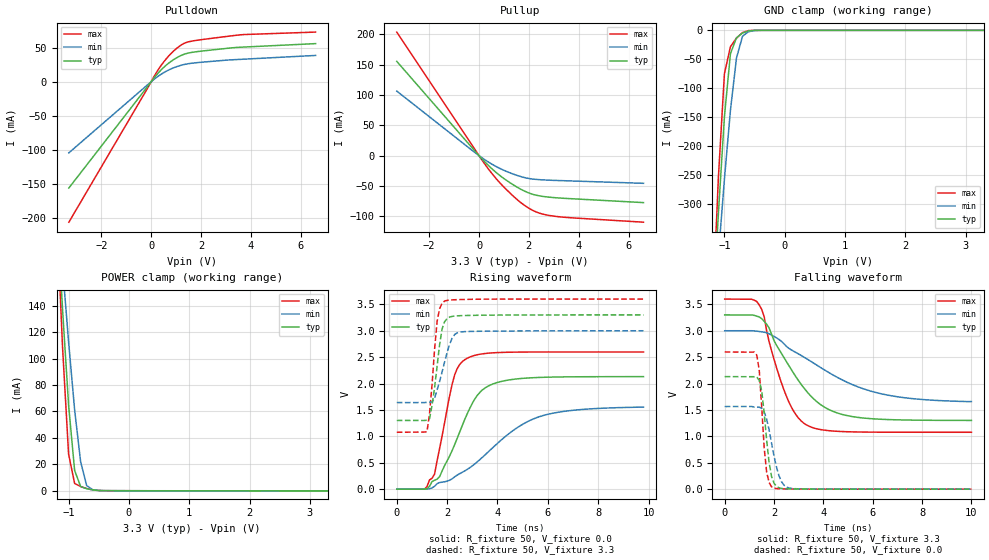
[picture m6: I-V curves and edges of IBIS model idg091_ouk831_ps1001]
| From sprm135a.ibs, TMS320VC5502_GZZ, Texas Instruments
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[Model]   idg091_ouk831_ps1001
Model_type   I/O
Vinh = 2.00
Vinl = 0.80
Enable   Active-Low
Polarity   Non-Inverting
| signals   A, GZ, Y
Vmeas = 1.5
|   typ   min   max
C_comp   1.997p   1.996p   1.999p
|   typ   min   max
[Temperature Range]   25   -40   125
|   typ   min   max
[Voltage Range]   3.30V   3.00V   3.60V
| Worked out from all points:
|   slope of the pulldown table from 0 to 0.495 V, typ, clamps not added: 24 ohm
|   slope of the pullup table from 0 to 0.495 V, typ, clamps not added: 23.8 ohm
|   GND clamp passes 1 mA (typ) near -0.60 V on its own axis
|   POWER clamp passes 1 mA (typ) near -0.64 V on its own axis
|   rising waveform, R_fixture 50, V_fixture 0.0: 20-80 % time 1.22ns typ, 2.49ns min, 657ps max; typ from 0 V to 2.13 V
|   falling waveform, R_fixture 50, V_fixture 3.3: 20-80 % time 1.7ns typ, 3.02ns min, 1.01ns max; typ from 3.3 V to 1.3 V
|   rising waveform, R_fixture 50, V_fixture 3.3: 20-80 % time 320ps typ, 466ps min, 257ps max; typ from 1.3 V to 3.3 V
|   falling waveform, R_fixture 50, V_fixture 0.0: 20-80 % time 292ps typ, 428ps min, 232ps max; typ from 2.13 V to 0 V
[Pulldown]
|   Voltage   I(typ)   I(min)   I(max)
-3.3V     -155.6mA   -104.1mA   -205.6mA
200mV     9.243mA    5.866mA    12.7mA
600mV     24.13mA    15.28mA    33.3mA
800mV     29.87mA    18.87mA    41.37mA
1.1V      36.63mA    23.02mA    51.08mA
1.3V      39.97mA    25.04mA    55.82mA
1.6V      42.83mA    27mA       59.29mA
3.5V      50.44mA    32.65mA    68.4mA
6.6V      55.87mA    38.54mA    72.75mA
[GND_clamp]
|   Voltage   I(typ)   I(min)   I(max)
-3.3V     -4.925A    -3.709A    -6.397A
-1.2V     -505.2mA   -529.5mA   -496.9mA
-1.1V     -317.2mA   -390.3mA   -254.5mA
-1V       -149.6mA   -257.7mA   -75.06mA
-900mV    -40.21mA   -138.1mA   -28.26mA
-800mV    -12.98mA   -47.92mA   -13.48mA
-700mV    -4.668mA   -10.2mA    -3.929mA
-600mV    -901.5uA   -2.361mA   -447.5uA
-400mV    -4.618uA   -50.5uA    -472.2nA
3.3V      444.1pA    1.932uA    266.4pA
[Pullup]
|   Voltage   I(typ)   I(min)   I(max)
-3.3V     155.5mA    106.5mA    203.9mA
-200mV    9.306mA    6.233mA    12.42mA
300mV     -13.07mA   -8.546mA   -17.75mA
600mV     -24.68mA   -16mA      -33.65mA
900mV     -34.78mA   -22.33mA   -47.64mA
1.4V      -48.81mA   -30.78mA   -67.77mA
1.7V      -55.9mA    -34.78mA   -78.19mA
2V        -61.53mA   -37.68mA   -86.71mA
2.3V      -65.31mA   -39.22mA   -93.01mA
2.9V      -68.83mA   -40.61mA   -99.22mA
3.7V      -71.03mA   -41.73mA   -102.5mA
6.6V      -77.46mA   -45.65mA   -109.8mA
[POWER_clamp]
|   Voltage   I(typ)   I(min)   I(max)
-3.3V     2.112A     1.593A     2.741A
-1.2V     218.1mA    229.3mA    213.2mA
-1.1V     137.3mA    169.6mA    108.5mA
-1V       64.88mA    112.7mA    27.71mA
-900mV    15.37mA    61.29mA    5.523mA
-800mV    3.157mA    21.76mA    3.151mA
-700mV    1.498mA    3.887mA    1.661mA
-600mV    649.7uA    748uA      624uA
-500mV    185.1uA    179.4uA    140.5uA
3.3V      -108.3uA   -68.12uA   -162.1uA
[Ramp]
|   I(typ)   I(min)   I(max)
dV/dt_r   1.278/1.218n   0.933/2.489n   1.559/0.652n
dV/dt_f   1.199/1.700n   0.806/3.024n   1.513/1.007n
[Rising Waveform]
R_fixture = 50
V_fixture = 0.0
|  pu_on
|  TIME   V(typ)   V(min)   V(max)
0s        5nV        18nV       4nV
1.1ns     50.37uV    -132uV     2.228mV
1.5ns     168.6mV    53.81mV    283.9mV
1.7ns     236mV      125mV      767.4mV
2.3ns     844.2mV    233.6mV    2.165V
2.8ns     1.429V     374.8mV    2.48V
3.2ns     1.777V     518.3mV    2.546V
3.7ns     1.968V     735.7mV    2.578V
5.6ns     2.115V     1.362V     2.597V
9.8ns     2.131V     1.554V     2.598V
[Falling Waveform]
R_fixture = 50
V_fixture = 3.3
V_fixture_min = 3.0
V_fixture_max = 3.6
|  pd_on
|  TIME   V(typ)   V(min)   V(max)
0s        3.3V       3V         3.6V
1.4ns     3.262V     2.986V     3.489V
1.6ns     3.179V     2.973V     3.268V
1.8ns     3.053V     2.942V     2.794V
2.5ns     2.417V     2.706V     1.761V
3.3ns     1.865V     2.476V     1.22V
4.1ns     1.538V     2.242V     1.114V
5.1ns     1.381V     1.995V     1.086V
7ns       1.313V     1.75V      1.078V
10ns      1.302V     1.659V     1.078V
[Rising Waveform]
R_fixture = 50
V_fixture = 3.3
V_fixture_min = 3.0
V_fixture_max = 3.6
|  pd_off
|  TIME   V(typ)   V(min)   V(max)
0s        1.301V     1.64V      1.078V
1.2ns     1.306V     1.644V     1.087V
1.3ns     1.333V     1.649V     1.429V
1.4ns     1.585V     1.648V     1.973V
1.6ns     2.321V     1.877V     3.172V
1.8ns     3.033V     2.218V     3.524V
1.9ns     3.172V     2.408V     3.562V
2.2ns     3.272V     2.86V      3.584V
2.5ns     3.285V     2.973V     3.591V
9.8ns     3.3V       3V         3.6V
[Falling Waveform]
R_fixture = 50
V_fixture = 0.0
|  pu_off
|  TIME   V(typ)   V(min)   V(max)
0s        2.131V     1.565V     2.598V
1.3ns     2.126V     1.554V     2.539V
1.4ns     2.059V     1.552V     2.255V
1.5ns     1.86V      1.531V     1.558V
1.6ns     1.446V     1.464V     786.2mV
1.7ns     930.2mV    1.329V     323.7mV
1.9ns     239.4mV    870.1mV    44.48mV
2.2ns     26.16mV    256.8mV    7.89mV
2.6ns     6.345mV    23.95mV    3.623mV
10ns      3.558uV    61.3uV     388nV
